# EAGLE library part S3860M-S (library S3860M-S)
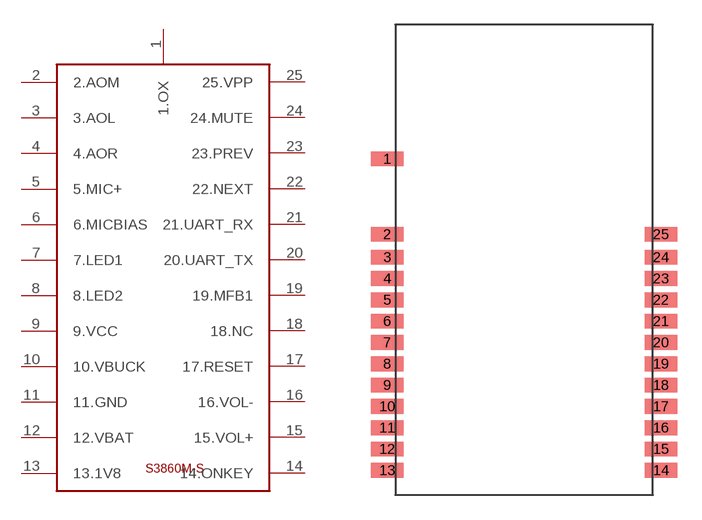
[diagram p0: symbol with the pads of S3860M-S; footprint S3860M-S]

Designator prefix -

## S3860M-S  [S3860M-S]
1  1.OX
2  2.AOM
3  3.AOL
4  4.AOR
5  5.MIC+
6  6.MICBIAS
7  7.LED1
8  8.LED2
9  9.VCC
10  10.VBUCK
11  11.GND
12  12.VBAT
13  13.1V8
14  14.ONKEY
15  15.VOL+
16  16.VOL-
17  17.RESET
18  18.NC
19  19.MFB1
20  20.UART_TX
21  21.UART_RX
22  22.NEXT
23  23.PREV
24  24.MUTE
25  25.VPP

## Footprint S3860M-S (pad centres in mm)
smd 2 x 0.9: 1 -0.5,-6.2; 2 -0.5,-10.8; 3 -0.5,-12.2; 4 -0.5,-13.5; 5 -0.5,-14.8; 6 -0.5,-16.1; 7 -0.5,-17.4; 8 -0.5,-18.7; 9 -0.5,-20; 10 -0.5,-21.3; 11 -0.5,-22.6; 12 -0.5,-23.9; 13 -0.5,-25.2; 14 16.2,-25.2; 15 16.2,-23.9; 16 16.2,-22.6; 17 16.2,-21.3; 18 16.2,-20; 19 16.2,-18.7; 20 16.2,-17.4; 21 16.2,-16.1; 22 16.2,-14.8; 23 16.2,-13.5; 24 16.2,-12.2; 25 16.2,-10.8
